| IBIS file stm32u375_385_ufbga100.ibs
[IBIS ver] 4.2
[File name] stm32u375_385_ufbga100.ibs
[File Rev] 1.2
[Date] 23-06-2025
[Source] Data Created at STMicroelectronics
[Notes]  File originated from ELDO simulations.
[Disclaimer]  This information is for modeling purpose only and is
   not guaranted. The information is subject to change without
   notice.
[Copyright] Copyright 2025 STMicroelectronics Inc.
|   Component stm32u375_385_ufbga100
[Component] stm32u375_385_ufbga100
[Manufacturer] STMicroelectronics
[Package]
| variable   typ   min   max
R_pkg  0  NA  NA
L_pkg  0  NA  NA
C_pkg  0  NA  NA
[Pin]   signal_name   model_name
A1  PE3  io8_ft_100m_hslv
A2  PE1  io8_ft_100m
A3  PB8  io8_ft_100m_hslv
A4  PH3-BOOT0  io8_ft_100m_hslv
A5  PD7  io8_ft_100m_hslv
A6  PD5  io8_ft_100m_hslv
A7  PB4  io8_ft_100m_hslv
A8  PB3  io8_ft_100m_hslv
A9  PA15  io8_ft_100m
A10  PA14  io8_ft_100m
A11  PA13  io8_ft_100m
A12  PA12  io8usb_ft_phy
B1  PE4  io8_ft_100m
B2  PE2  io8_ft_100m
B3  PB9  io8_ft_100m_hslv
B4  PB7  io8_ft_100m_hslv
B5  PB6  io8_ft_100m_hslv
B6  PD6  io8_ft_100m_hslv
B7  PD4  io8_ft_100m_hslv
B8  PD3  io8_ft_100m_hslv
B9  PD1  io8_ft_100m
B10  PC12  io8_ft_100m_hslv
B11  PC10  io8_ft_100m_hslv
B12  PA11  io8usb_ft_phy
C1  PC13  io8_ft_100m_v33
C2  PE5  io8_ft_100m
C3  PE0  io8_ft_100m
C4  VDD  power
C5  PB5  io8_ft_100m_hslv
C8  PD2  io8_ft_100m_hslv
C9  PD0  io8_ft_100m
C10  PC11  io8_ft_100m_hslv
C11  VDDUSB  power
C12  PA10  io8_ft_100m
D1  PC14-OSC32_IN  io_ft_tamp
D2  PE6  io8_ft_100m
D3  VSS  gnd
D10  PA9  io8_ft_100m
D11  PA8  io8_ft_100m_hslv
D12  PC9  io8_ft_100m_hslv
E1  PC15-OSC32_OUT  io_ft_tamp
E2  VBAT  power
E3  VSS  gnd
E10  PC8  io8_ft_100m_hslv
E11  PC7  io8_ft_100m_hslv
E12  PC6  io8_ft_100m_hslv
F1  PH0-OSC_IN  io8_ft_100m
F2  VSS  gnd
F11  VSS  gnd
F12  VSS  gnd
G1  PH1-OSC_OUT  io8_ft_100m
G2  VDD  power
G11  VDD  power
G12  VDD  power
H1  PC0  io8_ft_100m_hslv
H2  NRST  ioreset_v33
H3  VDD  power
H10  PD15  io8_ft_100m
H11  PD14  io8_ft_100m
H12  PD13  io8_ft_100m_hslv
J1  VSSA  nc
J2  PC1  io8_ft_100m_hslv
J3  PC2  io8_ft_100m_hslv
J10  PD12  io8_ft_100m_hslv
J11  PD11  io8_ft_100m
J12  PD10  io8_ft_100m
K1  VREFM  nc
K2  PC3  io8_ft_100m_hslv
K3  PA2  io8_ft_100m_hslv
K4  PA5  io8_ft_100m
K5  PC4  io8_ft_100m_hslv
K8  PD9  io8_ft_100m
K9  PD8  io8_ft_100m
K10  PB15  io8_ft_100m
K11  PB14  io8_ft_100m_hslv
K12  PB13  io8_ft_100m_hslv
L1  VREFP  nc
L2  PA0  io8_ft_100m
L3  PA3  io8_ft_100m_hslv
L4  PA6  io8_ft_100m_hslv
L5  PC5  io8_ft_100m
L6  PB2  io8_ft_100m_hslv
L7  PE8  io8_ft_100m
L8  PE10  io8_ft_100m_hslv
L9  PE12  io8_ft_100m_hslv
L10  PB10  io8_ft_100m_hslv
L11  VCAP  nc
L12  PB12  io8_ft_100m_hslv
M1  VDDA  nc
M2  PA1  io8_ft_100m_hslv
M3  PA4  io8_ft_100m_hslv
M4  PA7  io8_ft_100m_hslv
M5  PB0  io8_ft_100m_hslv
M6  PB1  io8_ft_100m_hslv
M7  PE7  io8_ft_100m
M8  PE9  io8_ft_100m_hslv
M9  PE11  io8_ft_100m_hslv
M10  PE13  io8_ft_100m_hslv
M11  PE14  io8_ft_100m_hslv
M12  PE15  io8_ft_100m_hslv
[Package Model]   454-ufbga-7x7-100-ldo-250417
[Pin Mapping]   pulldown_ref   pullup_ref   | Comment
A1  gndio  vddio
A2  gndio  vddio
A3  gndio  vddio
A4  gndio  vddio
A5  gndio  vddio
A6  gndio  vddio
A7  gndio  vddio
A8  gndio  vddio
A9  gndio  vddio
A10  gndio  vddio
A11  gndio  vddio
A12  gndio  vddusb  | Depending on IO usage
| A12  gndio  vddio  | Depending on IO usage
B1  gndio  vddio
B2  gndio  vddio
B3  gndio  vddio
B4  gndio  vddio
B5  gndio  vddio
B6  gndio  vddio
B7  gndio  vddio
B8  gndio  vddio
B9  gndio  vddio
B10  gndio  vddio
B11  gndio  vddio
B12  gndio  vddusb  | Depending on IO usage
| B12  gndio  vddio  | Depending on IO usage
C1  gndio  vsw
C2  gndio  vddio
C3  gndio  vddio
C4  nc  vddio
C5  gndio  vddio
C8  gndio  vddio
C9  gndio  vddio
C10  gndio  vddio
C11  nc  vddusb
C12  gndio  vddio
D1  gndio  vsw
D2  gndio  vddio
D3  gndio  nc
D10  gndio  vddio
D11  gndio  vddio
D12  gndio  vddio
E1  gndio  vsw
E2  nc  vsw
E3  gndio  nc
E10  gndio  vddio
E11  gndio  vddio
E12  gndio  vddio
F1  gndio  vddio
F2  gndio  nc
F11  gndio  nc
F12  gndio  nc
G1  gndio  vddio
G2  nc  vddio
G11  nc  vddio
G12  nc  vddio
H1  gndio  vddio
H2  gndio  vddio
H3  nc  vddio
H10  gndio  vddio
H11  gndio  vddio
H12  gndio  vddio
J1  nc  nc
J2  gndio  vddio
J3  gndio  vddio
J10  gndio  vddio
J11  gndio  vddio
J12  gndio  vddio
K1  nc  nc
K2  gndio  vddio
K3  gndio  vddio
K4  gndio  vddio
K5  gndio  vddio
K8  gndio  vddio
K9  gndio  vddio
K10  gndio  vddio
K11  gndio  vddio
K12  gndio  vddio
L1  nc  nc
L2  gndio  vddio
L3  gndio  vddio
L4  gndio  vddio
L5  gndio  vddio
L6  gndio  vddio
L7  gndio  vddio
L8  gndio  vddio
L9  gndio  vddio
L10  gndio  vddio
L11  nc  nc
L12  gndio  vddio
M1  nc  nc
M2  gndio  vddio
M3  gndio  vddio
M4  gndio  vddio
M5  gndio  vddio
M6  gndio  vddio
M7  gndio  vddio
M8  gndio  vddio
M9  gndio  vddio
M10  gndio  vddio
M11  gndio  vddio
M12  gndio  vddio
|[Diff Pin]  inv_pin  vdiff  tdelay_typ  tdelay_min  tdelay_max
|A12  B12  NA  NA  NA  NA
[Model Selector] io8_ft_100m
io8_ft_100m_ls_1v2  "GPIO 100MHz - 5V tolerant - low speed - 1.2V range"
io8_ft_100m_ls_1v8  "GPIO 100MHz - 5V tolerant - low speed - 1.8V range"
io8_ft_100m_ls_3v3  "GPIO 100MHz - 5V tolerant - low speed - 3.3V range"
io8_ft_100m_ms_1v2  "GPIO 100MHz - 5V tolerant - med speed - 1.2V range"
io8_ft_100m_ms_1v8  "GPIO 100MHz - 5V tolerant - med speed - 1.8V range"
io8_ft_100m_ms_3v3  "GPIO 100MHz - 5V tolerant - med speed - 3.3V range"
io8_ft_100m_fs_1v2  "GPIO 100MHz - 5V tolerant - fast speed - 1.2V range"
io8_ft_100m_fs_1v8  "GPIO 100MHz - 5V tolerant - fast speed - 1.8V range"
io8_ft_100m_fs_3v3  "GPIO 100MHz - 5V tolerant - fast speed - 3.3V range"
io8_ft_100m_hs_1v2  "GPIO 100MHz - 5V tolerant - high speed - 1.2V range"
io8_ft_100m_hs_1v8  "GPIO 100MHz - 5V tolerant - high speed - 1.8V range"
io8_ft_100m_hs_3v3  "GPIO 100MHz - 5V tolerant - high speed - 3.3V range"
[Model Selector] io8_ft_100m_hslv
io8_ft_100m_ls_1v2  "GPIO 100MHz - 5V tolerant - low speed - 1.2V range"
io8_ft_100m_ls_1v8  "GPIO 100MHz - 5V tolerant - low speed - 1.8V range"
io8_ft_100m_ls_3v3  "GPIO 100MHz - 5V tolerant - low speed - 3.3V range"
io8_ft_100m_ms_1v2  "GPIO 100MHz - 5V tolerant - med speed - 1.2V range"
io8_ft_100m_ms_1v8  "GPIO 100MHz - 5V tolerant - med speed - 1.8V range"
io8_ft_100m_ms_3v3  "GPIO 100MHz - 5V tolerant - med speed - 3.3V range"
io8_ft_100m_fs_1v2  "GPIO 100MHz - 5V tolerant - fast speed - 1.2V range"
io8_ft_100m_fs_1v8  "GPIO 100MHz - 5V tolerant - fast speed - 1.8V range"
io8_ft_100m_fs_3v3  "GPIO 100MHz - 5V tolerant - fast speed - 3.3V range"
io8_ft_100m_hs_1v2  "GPIO 100MHz - 5V tolerant - high speed - 1.2V range"
io8_ft_100m_hs_1v8  "GPIO 100MHz - 5V tolerant - high speed - 1.8V range"
io8_ft_100m_hs_3v3  "GPIO 100MHz - 5V tolerant - high speed - 3.3V range"
io8_ft_100m_hslv_ls_1v2  "GPIO 100MHz low voltage optimization - 5V tolerant - low speed - 1.2V range"
io8_ft_100m_hslv_ls_1v8  "GPIO 100MHz low voltage optimization - 5V tolerant - low speed - 1.8V range"
io8_ft_100m_hslv_ls_2v5  "GPIO 100MHz low voltage optimization - 5V tolerant - low speed - 3.3V range"
io8_ft_100m_hslv_ms_1v2  "GPIO 100MHz low voltage optimization - 5V tolerant - med speed - 1.2V range"
io8_ft_100m_hslv_ms_1v8  "GPIO 100MHz low voltage optimization - 5V tolerant - med speed - 1.8V range"
io8_ft_100m_hslv_ms_2v5  "GPIO 100MHz low voltage optimization - 5V tolerant - med speed - 3.3V range"
io8_ft_100m_hslv_fs_1v2  "GPIO 100MHz low voltage optimization - 5V tolerant - fast speed - 1.2V range"
io8_ft_100m_hslv_fs_1v8  "GPIO 100MHz low voltage optimization - 5V tolerant - fast speed - 1.8V range"
io8_ft_100m_hslv_fs_2v5  "GPIO 100MHz low voltage optimization - 5V tolerant - fast speed - 3.3V range"
io8_ft_100m_hslv_hs_1v2  "GPIO 100MHz low voltage optimization - 5V tolerant - high speed - 1.2V range"
io8_ft_100m_hslv_hs_1v8  "GPIO 100MHz low voltage optimization - 5V tolerant - high speed - 1.8V range"
io8_ft_100m_hslv_hs_2v5  "GPIO 100MHz low voltage optimization - 5V tolerant - high speed - 3.3V range"
[Model Selector] io8_ft_100m_v33
io8_ft_100m_v33_ls_1v2  "GPIO_V33 100MHz - 5V tolerant - low speed - 1.2V range"
io8_ft_100m_v33_ls_1v8  "GPIO_V33 100MHz - 5V tolerant - low speed - 1.8V range"
io8_ft_100m_v33_ls_3v3  "GPIO_V33 100MHz - 5V tolerant - low speed - 3.3V range"
io8_ft_100m_v33_ms_1v2  "GPIO_V33 100MHz - 5V tolerant - med speed - 1.2V range"
io8_ft_100m_v33_ms_1v8  "GPIO_V33 100MHz - 5V tolerant - med speed - 1.8V range"
io8_ft_100m_v33_ms_3v3  "GPIO_V33 100MHz - 5V tolerant - med speed - 3.3V range"
io8_ft_100m_v33_fs_1v2  "GPIO_V33 100MHz - 5V tolerant - fast speed - 1.2V range"
io8_ft_100m_v33_fs_1v8  "GPIO_V33 100MHz - 5V tolerant - fast speed - 1.8V range"
io8_ft_100m_v33_fs_3v3  "GPIO_V33 100MHz - 5V tolerant - fast speed - 3.3V range"
io8_ft_100m_v33_hs_1v2  "GPIO_V33 100MHz - 5V tolerant - high speed - 1.2V range"
io8_ft_100m_v33_hs_1v8  "GPIO_V33 100MHz - 5V tolerant - high speed - 1.8V range"
io8_ft_100m_v33_hs_3v3  "GPIO_V33 100MHz - 5V tolerant - high speed - 3.3V range"
[Model Selector] io8usb_ft_phy
io8_ft_100m_ls_1v2  "GPIO 100MHz - 5V tolerant - low speed - 1.2V range"
io8_ft_100m_ls_1v8  "GPIO 100MHz - 5V tolerant - low speed - 1.8V range"
io8_ft_100m_ls_3v3  "GPIO 100MHz - 5V tolerant - low speed - 3.3V range"
io8_ft_100m_ms_1v2  "GPIO 100MHz - 5V tolerant - med speed - 1.2V range"
io8_ft_100m_ms_1v8  "GPIO 100MHz - 5V tolerant - med speed - 1.8V range"
io8_ft_100m_ms_3v3  "GPIO 100MHz - 5V tolerant - med speed - 3.3V range"
io8_ft_100m_fs_1v2  "GPIO 100MHz - 5V tolerant - fast speed - 1.2V range"
io8_ft_100m_fs_1v8  "GPIO 100MHz - 5V tolerant - fast speed - 1.8V range"
io8_ft_100m_fs_3v3  "GPIO 100MHz - 5V tolerant - fast speed - 3.3V range"
io8_ft_100m_hs_1v2  "GPIO 100MHz - 5V tolerant - high speed - 1.2V range"
io8_ft_100m_hs_1v8  "GPIO 100MHz - 5V tolerant - high speed - 1.8V range"
io8_ft_100m_hs_3v3  "GPIO 100MHz - 5V tolerant - high speed - 3.3V range"
io8usb_ft_phy_hs_3v3   "USB full speed"
io8usb_ft_phy_ls_3v3   "USB low speed"
[Model Selector] io_ft_tamp
io_ft_tamp_ls_1v2 "io8_ft tamp low speed @ 1.2V"
io_ft_tamp_ls_1v8 "io8_ft tamp low speed @ 1.8V"
io_ft_tamp_ls_3v3 "io8_ft tamp low speed @ 3.3V"
io_ft_tamp_ms_1v2 "io8_ft tamp med speed @ 1.2V"
io_ft_tamp_ms_1v8 "io8_ft tamp med speed @ 1.8V"
io_ft_tamp_ms_3v3 "io8_ft tamp med speed @ 3.3V"
io_ft_tamp_fs_1v2 "io8_ft tamp fast speed @ 1.2V"
io_ft_tamp_fs_1v8 "io8_ft tamp fast speed @ 1.8V"
io_ft_tamp_fs_3v3 "io8_ft tamp fast speed @ 3.3V"
io_ft_tamp_hs_1v2 "io8_ft tamp high speed @ 1.2V"
io_ft_tamp_hs_1v8 "io8_ft tamp high speed @ 1.8V"
io_ft_tamp_hs_3v3 "io8_ft tamp high speed @ 3.3V"
[Model Selector] ioreset_v33
ioreset_v33_1v2 "Reset PAD. 5V tolerant. 1.2V range"
ioreset_v33_1v8 "Reset PAD. 5V tolerant. 1.8V range"
ioreset_v33_3v3 "Reset PAD. 5V tolerant. 3.3V range"
[Define Package Model]  454-ufbga-7x7-100-ldo-250417
[Manufacturer]  unknown
[OEM]  unknown
[Description]  unknown
[Number Of Pins]  92
[Pin Numbers]
| Pin Name Terminal   Net Name   Starting Node   Ending Node
H2 | NRST
L2 | PA0
M2 | PA1
K3 | PA2
L3 | PA3
M3 | PA4
K4 | PA5
L4 | PA6
M4 | PA7
D11 | PA8
D10 | PA9
C12 | PA10
B12 | PA11
A12 | PA12
A11 | PA13
A10 | PA14
A9 | PA15
M5 | PB0
M6 | PB1
L6 | PB2
A8 | PB3
A7 | PB4
C5 | PB5
B5 | PB6
B4 | PB7
A3 | PB8
B3 | PB9
L10 | PB10
L12 | PB12
K12 | PB13
K11 | PB14
K10 | PB15
H1 | PC0
J2 | PC1
J3 | PC2
K2 | PC3
K5 | PC4
L5 | PC5
E12 | PC6
E11 | PC7
E10 | PC8
D12 | PC9
B11 | PC10
C10 | PC11
B10 | PC12
C1 | PC13
D1 | PC14-OSC32_IN
E1 | PC15-OSC32_OUT
C9 | PD0
B9 | PD1
C8 | PD2
B8 | PD3
B7 | PD4
A6 | PD5
B6 | PD6
A5 | PD7
K9 | PD8
K8 | PD9
J12 | PD10
J11 | PD11
J10 | PD12
H12 | PD13
H11 | PD14
H10 | PD15
C3 | PE0
A2 | PE1
B2 | PE2
A1 | PE3
B1 | PE4
C2 | PE5
D2 | PE6
M7 | PE7
L7 | PE8
M8 | PE9
L8 | PE10
M9 | PE11
L9 | PE12
M10 | PE13
M11 | PE14
M12 | PE15
F1 | PH0-OSC_IN
G1 | PH1-OSC_OUT
A4 | PH3-BOOT0
E2 | VBAT
L11 | VCAP
C4 | VDD
M1 | VDDA
C11 | VDDUSB
K1 | VREFM
L1 | VREFP
D3 | VSS
J1 | VSSA
|[Merged Pins]  C4
|G2  |  VDD
|G11  |  VDD
|G12  |  VDD
|H3  |  VDD
|[Merged Pins]  D3
|E3  |  VSS
|F2  |  VSS
|F11  |  VSS
|F12  |  VSS
[Model Data]
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[End Model Data]
[End Package Model]
|End [Component]
| Models and submodels in the file (53): io8_ft_100m_fs_1v2 (I/O), io8_ft_100m_fs_1v8 (I/O), io8_ft_100m_fs_3v3 (I/O), io8_ft_100m_hs_1v2 (I/O), io8_ft_100m_hs_1v8 (I/O), io8_ft_100m_hs_3v3 (I/O), io8_ft_100m_hslv_fs_1v2 (I/O), io8_ft_100m_hslv_fs_1v8 (I/O), io8_ft_100m_hslv_fs_2v5 (I/O), io8_ft_100m_hslv_hs_1v2 (I/O), io8_ft_100m_hslv_hs_1v8 (I/O), io8_ft_100m_hslv_hs_2v5 (I/O), io8_ft_100m_hslv_ls_1v2 (I/O), io8_ft_100m_hslv_ls_1v8 (I/O), io8_ft_100m_hslv_ls_2v5 (I/O), io8_ft_100m_hslv_ms_1v2 (I/O), io8_ft_100m_hslv_ms_1v8 (I/O), io8_ft_100m_hslv_ms_2v5 (I/O), io8_ft_100m_ls_1v2 (I/O), io8_ft_100m_ls_1v8 (I/O), io8_ft_100m_ls_3v3 (I/O), io8_ft_100m_ms_1v2 (I/O), io8_ft_100m_ms_1v8 (I/O), io8_ft_100m_ms_3v3 (I/O), io8_ft_100m_v33_fs_1v2 (I/O), io8_ft_100m_v33_fs_1v8 (I/O), io8_ft_100m_v33_fs_3v3 (I/O), io8_ft_100m_v33_hs_1v2 (I/O), io8_ft_100m_v33_hs_1v8 (I/O), io8_ft_100m_v33_hs_3v3 (I/O), io8_ft_100m_v33_ls_1v2 (I/O), io8_ft_100m_v33_ls_1v8 (I/O), io8_ft_100m_v33_ls_3v3 (I/O), io8_ft_100m_v33_ms_1v2 (I/O), io8_ft_100m_v33_ms_1v8 (I/O), io8_ft_100m_v33_ms_3v3 (I/O), io8usb_ft_phy_hs_3v3 (I/O), io8usb_ft_phy_ls_3v3 (I/O), io_ft_tamp_fs_1v2 (I/O), io_ft_tamp_fs_1v8 (I/O), io_ft_tamp_fs_3v3 (I/O), io_ft_tamp_hs_1v2 (I/O), io_ft_tamp_hs_1v8 (I/O), io_ft_tamp_hs_3v3 (I/O), io_ft_tamp_ls_1v2 (I/O), io_ft_tamp_ls_1v8 (I/O), io_ft_tamp_ls_3v3 (I/O), io_ft_tamp_ms_1v2 (I/O), io_ft_tamp_ms_1v8 (I/O), io_ft_tamp_ms_3v3 (I/O), ioreset_v33_1v2 (I/O_open_drain), ioreset_v33_1v8 (I/O_open_drain), ioreset_v33_3v3 (I/O_open_drain)
